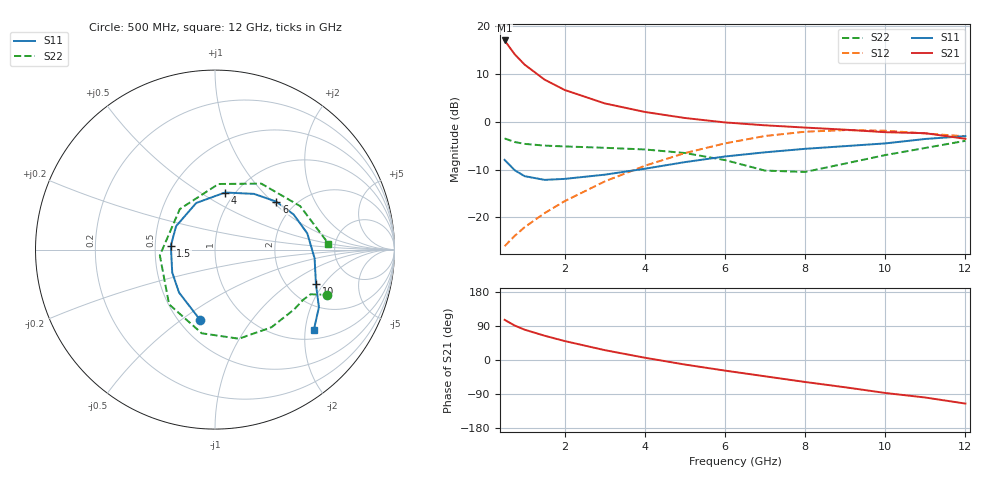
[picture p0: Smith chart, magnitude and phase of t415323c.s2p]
!AT-41532
!S-PARAMETERS at Vce=2.7V  Ic=5mA.  LAST UPDATED 05-29-98
# ghz s ma r 50
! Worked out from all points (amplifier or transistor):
!   15 points, 500 MHz to 12 GHz, reference 50 ohm
!   highest |S21| = 17.0 dB at 500 MHz (marker M1)
!   |S21| within 3 dB of that: start of sweep to 763.8 MHz
!   unconditionally stable (mu >= 1): 984 MHz to 2.334 GHz
!   at 1 GHz: K = 1.01, MAG = 16.5 dB, |S12| = -22.0 dB
!   at 5 GHz: K = 0.81, MSG = 3.7 dB, |S12| = -6.5 dB
!   at 12 GHz: K = 1.00, MSG = -0.3 dB, |S12| = -3.0 dB
!   lowest NFmin = 1.20 dB at 900 MHz
!   S11 on the Smith chart (normalised r, x): 500 MHz: 0.63, -0.59; 1.5 GHz: 0.60, +0.03; 4 GHz: 0.90, +0.64; 6 GHz: 1.61, +1.06; 10 GHz: 2.82, -1.69; 12 GHz: 1.24, -2.23
0.5  0.4 -102.0  7.106 106.0  0.05 59.0  0.671 -22.0
0.75  0.312 -130.0  5.101 91.0  0.064 60.0  0.615 -24.0
1  0.27 -152.0  3.969 80.0  0.079 61.0  0.588 -25.0
1.5  0.247 175.0  2.762 64.0  0.111 63.0  0.564 -30.0
2  0.253 149.0  2.154 50.0  0.148 62.0  0.553 -37.0
3  0.28 112.0  1.559 26.0  0.238 55.0  0.535 -54.0
4  0.323 80.0  1.269 6.0  0.347 43.0  0.514 -75.0
5  0.379 55.0  1.097 -12.0  0.471 27.0  0.472 -99.0
6  0.434 38.0  0.986 -28.0  0.595 9.0  0.398 -130.0
7  0.48 24.0  0.92 -43.0  0.711 -11.0  0.309 -174.0
8  0.522 10.0  0.871 -58.0  0.788 -32.0  0.299 131.0
9  0.557 -5.0  0.828 -72.0  0.82 -53.0  0.366 87.0
10  0.595 -19.0  0.779 -87.0  0.808 -73.0  0.449 55.0
11  0.662 -29.0  0.761 -99.0  0.756 -92.0  0.533 27.0
12  0.709 -39.0  0.664 -115.0  0.705 -107.0  0.633 3.0
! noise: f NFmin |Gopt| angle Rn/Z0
0.9  1.2  0.283  106  0.15
1.8  1.4  0.41  -165  0.08
2  1.5  0.44  -151  0.1
2.5  1.7  0.53  -126  0.18
3  1.9  0.6  -106  0.37
3.5  2.2  0.67  -86  0.7
4  2.5  0.71  -69  1.16
